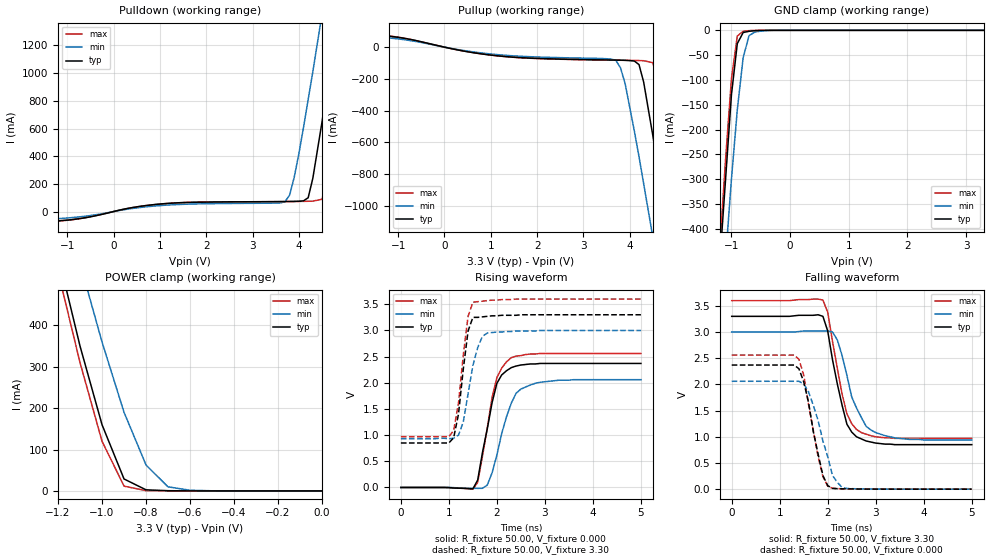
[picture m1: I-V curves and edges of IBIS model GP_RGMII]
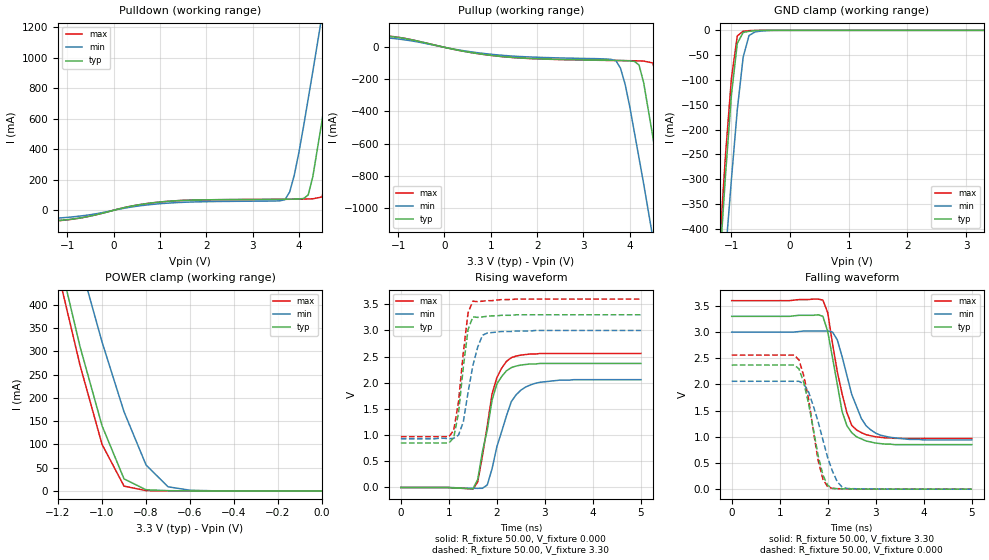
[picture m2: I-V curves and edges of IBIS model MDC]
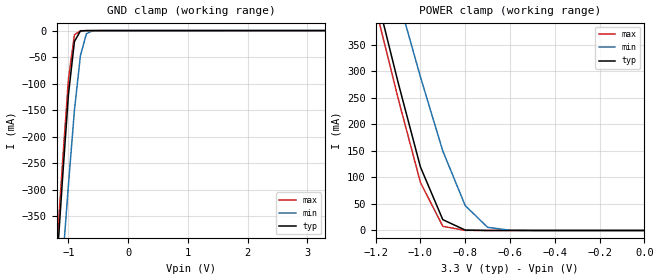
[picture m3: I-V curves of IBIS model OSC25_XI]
|   National Semiconductor Corporation
|   Networks Division
|   IBIS Model for DP83865
|   128 Pin PQFP Package
| IBIS file DP83865.ibs was created using s2ibis2 version 2.1
| North Carolina State University Electronics Research Laboratory 1997
| http://www.eigroup.org/ibis/tools.htm -> SPICE-toIBISconversion(IBISv2.1)
| s2ibis2.tar.Z   11FEB97   652K
| s2ibis2_fix.tar.Z 13MAY97   119K
[IBIS ver]   3.2
[File name]   dp83865.ibs
[File Rev]   1.0
[Date]   07MAY04
[Source]   National Semiconductor Corporation, Networks Division
[Notes]   For questions or comments contact
   jeff.zhang@nsc.com
   Spectre s2ibis simulations, created by Jeff Zhang.
| Due to IBIS modeling limitations and design complexity this model
| does not support the Ethernet Transmit Data pins:
| [Pin]   signal_name   model_name
|108   MDIA_P   NC
|109   MDIA_N   NC
|114   MDIB_P   NC
|115   MDIB_N   NC
|120   MDIC_P   NC
|121   MDIC_N   NC
|126   MDID_P   NC
|127   MDID_N   NC
| Please refer to product datasheet and application notes for PC board
| layout recommendations.
[Disclaimer]  Absolutely no guarantees, for modeling purposes only.
   National Semiconductor Corporation hereby grants the user of this IBIS
model a non-exclusive, nontransferable license to use this IBIS model under
the following terms. Before using this IBIS model, the user should read this
license.  If the user does not accept these terms,  the IBIS model should be
returned to National within 30 days.
   The user is granted this license only to use the IBIS model and is not
granted rights to sell, load, rent, lease or license the IBIS model in whole
or in part, or in modified form to anyone other than user. User may modify
the IBIS model to suit its specific applications but rights to derivative
works and such modifications shall belong to National.
   This IBIS model is provided on an "AS IS" basis and National makes
absolutely no warranty with respect to the information contained herein.
NATIONAL DISCLAIMS AND CUSTOMER WAIVES ALL WARRANTIES, EXPRESS OR IMPLIED,
INCLUDING WARRANTIES OF MERCHANTABILITY OR FITNESS FOR A PARTICULAR PURPOSE.
The entire risk as to quality and performance is with the Customer.
ACCORDINGLY, IN NO EVENT SHALL THE COMPANY BE LIABLE FOR ANY DAMAGES, WHETHER
IN CONTRACT OR COURT, INCLUDING ANY LOST PROFITS OR OTHER INCIDENTAL,
CONSEQUENTIAL, EXEMPLARY, OR PUNITIVE DAMAGES ARISING OUT OF THE USE OR
APPLICATION OF THE IBIS model provided in this package. Further, National
reserves the right to make changes without notice to any product herein to
improve reliability, function, or design. National does not convey any license
under patent rights or any other intellectual property rights, including those
of third parties.
   National is not obligated to provide maintenance or support
for the licensed IBIS model.
[Copyright]   Copyright 2001, National Semiconductor Corporation, All rights
   reserved
|   Component DP83865
[Component]   DP83865
[Manufacturer]   National Semiconductor Corporation
[Package]
| variable   typ   min   max
R_pkg   0.230   0.113   0.305
L_pkg   7.507nH   4.865nH   9.669nH
C_pkg   1.044pF   0.511pF   1.471pF
[Pin]  signal_name   model_name   R_pin   L_pin   C_pin
1   NON_IEEE   GP_RGMII   0.253   9.370nH   1.083pF
2   RESERVED   GP_RGMII   0.255   9.000nH   1.468pF
3   INTERRUPT   GP_RGMII   0.254   8.684nH   1.388pF
4   IO_VDD   POWER   0.255   8.476nH   1.373pF
5   VSS   GND   0.150   6.714nH   1.391pF
6   TX_TCLK   GP_RGMII   0.247   8.104nH   0.756pF
7   ACTIVITY_LED   GP_RGMII   0.246   7.817nH   1.158pF
8   LINK10_LED   GP_RGMII   0.144   6.090nH   1.163pF
9   LINK100_LED   GP_RGMII   0.240   7.452nH   1.064pF
10   AN_EN   GP_RGMII   0.238   7.286nH   1.020pF
11   CORE_VDD   POWER   0.248   7.324nH   0.972pF
12   VSS   GND   0.139   5.513nH   1.007pF
13   PHYADDR0   GP_RGMII   0.241   6.994nH   0.903pF
14   PHYADDR1   GP_RGMII   0.239   6.852nH   0.861pF
15   IO_VDD   POWER   0.236   6.751nH   0.826pF
16   VSS   GND   0.132   5.054nH   0.863pF
17   PHYADDR2   GP_RGMII   0.235   6.563nH   0.771pF
18   PHYADDR3   GP_RGMII   0.235   6.493nH   0.758pF
19   CORE_VDD   POWER   0.236   6.496nH   0.747pF
20   VSS   GND   0.131   4.865nH   0.830pF
21   IO_VDD   POWER   0.234   6.478nH   0.779pF
22   VSS   GND   0.130   4.931nH   0.841pF
23   RESERVED   RGMII125   0.233   6.607nH   0.798pF
24   TCK   RGMII125   0.233   6.664nH   0.510pF
25   CORE_VDD   POWER   0.230   6.679nH   0.854pF
26   VSS   GND   0.131   5.237nH   0.959pF
27   TMS   RGMII125   0.230   6.897nH   0.933pF
28   TDO   RGMII125   0.231   7.040nH   0.965pF
29   IO_VDD   POWER   0.233   7.185nH   1.016pF
30   VSS   GND   0.138   5.850nH   1.124pF
31   TDI   RGMII125   0.237   7.512nH   1.094pF
32   TRST   RGMII125   0.240   7.696nH   1.153pF
33   RESET   RGMII125   0.242   7.992nH   1.236pF
34   VDD_SEL_   POWER   0.249   8.221nH   1.314pF
35   CORE_VDD   POWER   0.255   8.455nH   1.368pF
36   VSS   GND   0.154   7.133nH   1.451pF
37   IO_VDD   POWER   0.255   8.994nH   1.467pF
38   VSS   GND   0.153   7.819nH   1.139pF
39   COL   RGMII125   0.269   9.342nH   0.946pF
40   CRS/RGMII_SEL1 RGMII125   0.263   8.929nH   1.261pF
41   RX_ER   RGMII125   0.259   8.740nH   1.215pF
42   IO_VDD   POWER   0.256   8.546nH   1.164pF
43   VSS   GND   0.146   6.880nH   1.200pF
44   RX_DV   RGMII125   0.257   8.489nH   1.110pF
45   RXD7   RGMII125   0.257   8.359nH   1.082pF
46   RXD6   RGMII125   0.257   8.221nH   1.043pF
47   RXD5   RGMII125   0.259   8.168nH   0.992pF
48   CORE_VDD   POWER   0.261   8.113nH   1.023pF
49   VSS   GND   0.150   6.313nH   1.095pF
50   RXD4   RGMII125   0.268   8.069nH   0.982pF
51   RXD3   RGMII125   0.270   7.874nH   1.019pF
52   RXD2   RGMII125   0.271   7.932nH   1.006pF
53   IO_VDD   POWER   0.266   7.939nH   0.969pF
54   VSS   GND   0.147   6.100nH   1.046pF
55   RXD1   RGMII125   0.260   7.942nH   0.987pF
56   RXD0   RGMII125   0.258   7.994nH   1.009pF
57   RX_CLK   RGMII125   0.258   8.084nH   1.038pF
58   IO_VDD   POWER   0.257   8.189nH   1.069pF
59   VSS   GND   0.147   6.592nH   1.176pF
60   TX_CLK   RGMII125   0.257   8.416nH   1.131pF
61   TX_ER   RGMII125   0.259   8.605nH   1.166pF
62   TX_EN   RGMII125   0.262   8.804nH   1.217pF
63   CORE_VDD   POWER   0.266   9.075nH   1.269pF
64   VSS   GND   0.158   7.609nH   1.020pF
65   TXD7   RGMII125   0.249   9.245nH   1.078pF
66   TXD6   RGMII125   0.251   8.879nH   1.471pF
67   TXD5   RGMII125   0.250   8.587nH   1.388pF
68   TXD4   RGMII125   0.250   8.299nH   1.374pF
69   IO_VDD   POWER   0.245   8.062nH   1.319pF
70   VSS   GND   0.144   6.356nH   1.297pF
71   TXD3   RGMII125   0.238   7.661nH   1.152pF
72   TXD2   RGMII125   0.236   7.480nH   1.092pF
73   CORE_VDD   POWER   0.232   7.306nH   1.059pF
74   VSS   GND   0.135   5.664nH   1.077pF
75   TXD1   RGMII125   0.230   7.022nH   0.964pF
76   TXD0   RGMII125   0.230   6.884nH   0.932pF
77   IO_VDD   POWER   0.234   6.820nH   0.895pF
78   VSS   GND   0.132   5.152nH   0.920pF
79   GTX_CLK   RGMII125   0.234   6.685nH   0.823pF
80   MDIO   MDC   0.234   6.607nH   0.792pF
81   MDC   MDC   0.233   6.528nH   0.770pF
82   VSS   GND   0.234   6.473nH   0.757pF
83   IO_VDD   POWER   0.236   6.484nH   0.747pF
84   RESERVED   RGMII125   0.244   6.522nH   0.764pF
85   CLK_TO_MAC   RGMII125   0.234   6.472nH   0.779pF
86   CLK_IN   OSC25_XI   0.234   6.563nH   0.774pF
87   CLK_OUT   GP_RGMII   0.234   6.659nH   0.800pF
88   MAC_CLK_EN   GP_RGMII   0.234   6.756nH   0.514pF
89   MDIX_EN   GP_RGMII   0.238   6.847nH   0.860pF
90   IO_VDD   POWER   0.239   6.970nH   0.903pF
91   VSS   GND   0.139   5.546nH   1.010pF
92   CORE_VDD   POWER   0.244   7.313nH   0.975pF
93   VSS   GND   0.144   5.860nH   1.094pF
94   MULTI_EN   GP_RGMII   0.244   7.545nH   1.068pF
95   PHYADDR4   GP_RGMII   0.248   7.698nH   1.099pF
96   AFE_VDD   POWER   0.242   7.744nH   1.155pF
97   VSS   GND   0.241   7.925nH   1.237pF
98   PGM_VDD   POWER   0.247   8.077nH   1.314pF
99   VSS   GND   0.250   8.273nH   1.366pF
100   CORE_VDD   POWER   0.251   8.509nH   1.382pF
101   BG_VDD   POWER   0.251   8.799nH   1.464pF
102   BG_REF   POWER   0.247   9.140nH   1.069pF
103   RX_VDD   POWER   0.287   9.669nH   0.956pF
104   VSS   GND   0.280   9.261nH   1.272pF
105   RX_VDD   POWER   0.275   9.149nH   1.222pF
106   VSS   GND   0.270   8.650nH   1.140pF
107   VSS   GND   0.210   7.942nH   1.078pF
108   MDIA_P   NC   0.287   8.392nH   1.028pF
109   MDIA_N   NC   0.285   8.215nH   0.983pF
110   VSS   GND   0.121   6.271nH   1.022pF
111   RX_VDD   POWER   0.286   8.048nH   0.940pF
112   VSS   GND   0.287   7.943nH   0.901pF
113   VSS   GND   0.191   7.185nH   0.874pF
114   MDIB_P   NC   0.292   7.844nH   0.878pF
115   MDIB_N   NC   0.305   7.848nH   0.928pF
116   VSS   GND   0.113   5.862nH   0.962pF
117   RX_VDD   POWER   0.291   7.804nH   0.868pF
118   VSS   GND   0.287   7.791nH   0.897pF
119   VSS   GND   0.189   7.158nH   0.916pF
120   MDIC_P   NC   0.282   7.898nH   0.939pF
121   MDIC_N   NC   0.281   7.966nH   0.968pF
122   VSS   GND   0.117   6.202nH   1.059pF
123   RX_VDD   POWER   0.280   8.214nH   1.022pF
124   VSS   GND   0.282   8.370nH   1.054pF
125   VSS   GND   0.208   7.942nH   1.125pF
126   MDID_P   NC   0.288   8.769nH   1.145pF
127   MDID_N   NC   0.293   9.013nH   1.224pF
128   VSS   GND   0.140   7.489nH   1.013pF
| Models and submodels in the file (4): GP_RGMII (I/O), MDC (I/O), OSC25_XI (Input), RGMII125 (I/O)
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|   Model GP_RGMII
[Model]   GP_RGMII
Model_type   I/O
Polarity   Non-Inverting
Enable   Active-High
Vinl =   0.80V
Vinh =   2.00V
Vmeas =   1.50V
Cref =  20.00pF
Rref = 100.00k
C_comp   5.00pF   5.00pF   5.00pF
[Temperature Range]   25.00   0.14k   0.000
[Voltage Range]   3.30V   3.00V   3.60V
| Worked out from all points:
|   slope of the pulldown table from 0 to 0.495 V, typ, clamps not added: 14.7 ohm
|   slope of the pullup table from 0 to 0.495 V, typ, clamps not added: 17.2 ohm
|   GND clamp passes 1 mA (typ) near -0.62 V on its own axis
|   POWER clamp passes 1 mA (typ) near -0.72 V on its own axis
|   rising waveform, R_fixture 50.00, V_fixture 0.000: 20-80 % time 312ps typ, 381ps min, 304ps max; typ from 0 V to 2.37 V
|   rising waveform, R_fixture 50.00, V_fixture 3.30: 20-80 % time 189ps typ, 258ps min, 195ps max; typ from 0.85 V to 3.3 V
|   falling waveform, R_fixture 50.00, V_fixture 3.30: 20-80 % time 334ps typ, 423ps min, 330ps max; typ from 3.3 V to 0.85 V
|   falling waveform, R_fixture 50.00, V_fixture 0.000: 20-80 % time 308ps typ, 376ps min, 305ps max; typ from 2.37 V to 0 V
[Pulldown]
| voltage   I(typ)   I(min)   I(max)
-3.3V     -89.91mA   -76.56mA   -93.13mA
-1V       -61.93mA   -46.66mA   -63.1mA
1.2V      59.47mA    47.45mA    59.1mA
3.7V      72.36mA    71.01mA    71.87mA
3.9V      73.37mA    250mA      72.58mA
4.2V      100mA      810mA      74.31mA
4.3V      240mA      1.01A      75.21mA
4.5V      650mA      1.43A      88.74mA
4.7V      1.11A      1.86A      390mA
4.9V      1.58A      2.29A      840mA
5.1V      2.07A      2.73A      1.32A
6.6V      5.81A      6.08A      5.12A
[Pullup]
| voltage   I(typ)   I(min)   I(max)
-3.3V     100mA      91.31mA    110mA
-1.5V     79.4mA     67.53mA    81.97mA
1.3V      -58.96mA   -51mA      -59.25mA
3.7V      -81.52mA   -83.17mA   -82.27mA
3.9V      -83.1mA    -230mA     -83.06mA
4.2V      -110mA     -690mA     -84.55mA
4.3V      -220mA     -860mA     -85.63mA
4.5V      -560mA     -1.2A      -97.98mA
4.7V      -940mA     -1.55A     -350mA
4.9V      -1.33A     -1.91A     -720mA
5.1V      -1.73A     -2.27A     -1.12A
6.6V      -4.89A     -5.08A     -4.33A
[GND_clamp]
| voltage   I(typ)   I(min)   I(max)
-3.3V     -4.64A     -4.34A     -4.71A
-1.2V     -470mA     -620mA     -440mA
-1.1V     -300mA     -460mA     -260mA
-1V       -130mA     -300mA     -97.76mA
-900mV    -26.77mA   -160mA     -11.53mA
-800mV    -4.41mA    -54.89mA   -1.88mA
-700mV    -1.97mA    -10.78mA   -630uA
-600mV    -770uA     -3.36mA    -120uA
-500mV    -170uA     -1.53mA    -11.66uA
-200mV    -41.48nA   -16.34uA   -940pA
3.3V      180pA      10.43uA    45.9pA
[POWER_clamp]
| voltage   I(typ)   I(min)   I(max)
-3.3V     5.63A      5.27A      5.71A
-1.2V     570mA      750mA      530mA
-1.1V     350mA      550mA      310mA
-1V       160mA      360mA      120mA
-900mV    28.86mA    190mA      11.54mA
-800mV    2.64mA     62.61mA    730uA
-700mV    550uA      9.86mA     87.59uA
-600mV    98.75uA    1.62mA     9.39uA
0V        180pA      380nA      53.88pA
[Ramp]
| variable   typ   min   max
dV/dt_r   1.92/0.12n   1.74/0.15n   2.09/0.12n
dV/dt_f   1.93/99.31p   1.74/0.12n   2.11/0.10n
R_load = 0.50k
[Rising Waveform]
R_fixture = 50.00
V_fixture = 0.000
V_fixture_min = 0.000
V_fixture_max = 0.000
| time   V(typ)   V(min)   V(max)
0s        1.26nV     480nV      1.01nV
1.5ns     -26.8mV    -15.77mV   -32.46mV
1.6ns     140mV      -17.36mV   96.56mV
1.8ns     1.12V      45.67mV    1.14V
1.9ns     1.62V      280mV      1.72V
2ns       1.99V      620mV      2.1V
2.3ns     2.29V      1.61V      2.48V
2.5ns     2.34V      1.88V      2.52V
2.9ns     2.37V      2.01V      2.56V
5ns       2.37V      2.06V      2.56V
[Rising Waveform]
R_fixture = 50.00
V_fixture = 3.30
V_fixture_min = 3.00
V_fixture_max = 3.60
| time   V(typ)   V(min)   V(max)
0s        850mV      930mV      970mV
1ns       850mV      930mV      970mV
1.1ns     950mV      940mV      1.09V
1.2ns     1.4V       1V         1.61V
1.3ns     2.26V      1.25V      2.53V
1.4ns     2.99V      1.79V      3.27V
1.5ns     3.25V      2.33V      3.54V
1.7ns     3.26V      2.89V      3.56V
1.8ns     3.27V      2.95V      3.57V
5ns       3.3V       3V         3.6V
[Falling Waveform]
R_fixture = 50.00
V_fixture = 3.30
V_fixture_min = 3.00
V_fixture_max = 3.60
| time   V(typ)   V(min)   V(max)
0s        3.3V       3V         3.6V
1.9ns     3.3V       3.02V      3.61V
2ns       3.02V      3.02V      3.38V
2.2ns     2.01V      2.85V      2.31V
2.4ns     1.24V      2.17V      1.44V
2.5ns     1.09V      1.76V      1.25V
2.7ns     960mV      1.37V      1.08V
2.9ns     900mV      1.13V      1.02V
3.4ns     850mV      980mV      970mV
5ns       850mV      940mV      970mV
[Falling Waveform]
R_fixture = 50.00
V_fixture = 0.000
V_fixture_min = 0.000
V_fixture_max = 0.000
| time   V(typ)   V(min)   V(max)
0s        2.37V      2.06V      2.56V
1.4ns     2.3V       2.06V      2.48V
1.5ns     2.05V      2.01V      2.18V
1.6ns     1.66V      1.86V      1.62V
1.8ns     670mV      1.31V      620mV
1.9ns     260mV      920mV      240mV
2ns       67.8mV     620mV      57.17mV
2.1ns     15.64mV    260mV      16.13mV
2.3ns     6.95mV     32.77mV    7.28mV
5ns       -110nV     14.23uV    1.22uV
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|   Model MDC
[Model]   MDC
Model_type   I/O
Polarity   Non-Inverting
Enable   Active-High
Vinl =   0.80V
Vinh =   2.00V
Vmeas =   1.50V
Cref =  20.00pF
Rref = 100.00k
C_comp   5.00pF   5.00pF   5.00pF
[Temperature Range]   25.00   0.14k   0.000
[Voltage Range]   3.30V   3.00V   3.60V
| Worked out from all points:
|   slope of the pulldown table from 0 to 0.495 V, typ, clamps not added: 14.7 ohm
|   slope of the pullup table from 0 to 0.495 V, typ, clamps not added: 17.2 ohm
|   GND clamp passes 1 mA (typ) near -0.62 V on its own axis
|   POWER clamp passes 1 mA (typ) near -0.72 V on its own axis
|   rising waveform, R_fixture 50.00, V_fixture 0.000: 20-80 % time 313ps typ, 394ps min, 302ps max; typ from 0 V to 2.37 V
|   rising waveform, R_fixture 50.00, V_fixture 3.30: 20-80 % time 188ps typ, 257ps min, 190ps max; typ from 0.85 V to 3.3 V
|   falling waveform, R_fixture 50.00, V_fixture 3.30: 20-80 % time 312ps typ, 417ps min, 340ps max; typ from 3.3 V to 0.85 V
|   falling waveform, R_fixture 50.00, V_fixture 0.000: 20-80 % time 309ps typ, 394ps min, 283ps max; typ from 2.37 V to 0 V
[Pulldown]
| voltage   I(typ)   I(min)   I(max)
-3.3V     -89.91mA   -76.56mA   -93.13mA
-1V       -61.93mA   -46.66mA   -63.1mA
1.2V      59.47mA    47.45mA    59.1mA
3.7V      72.36mA    69.99mA    71.87mA
3.9V      73.37mA    230mA      72.58mA
4.2V      100mA      730mA      74.31mA
4.3V      220mA      910mA      75.21mA
4.5V      590mA      1.28A      87.5mA
4.7V      1A         1.66A      350mA
4.9V      1.42A      2.04A      760mA
5.1V      1.85A      2.43A      1.19A
6.6V      5.19A      5.43A      4.58A
[Pullup]
| voltage   I(typ)   I(min)   I(max)
-3.3V     100mA      91.31mA    110mA
-1.5V     79.4mA     67.53mA    81.97mA
1.3V      -58.96mA   -51mA      -59.25mA
3.7V      -81.52mA   -82.85mA   -82.27mA
3.9V      -83.1mA    -230mA     -83.06mA
4.2V      -110mA     -690mA     -84.55mA
4.3V      -220mA     -850mA     -85.62mA
4.5V      -560mA     -1.19A     -97.65mA
4.7V      -930mA     -1.54A     -340mA
4.9V      -1.32A     -1.89A     -720mA
5.1V      -1.71A     -2.25A     -1.11A
6.6V      -4.85A     -5.04A     -4.3A
[GND_clamp]
| voltage   I(typ)   I(min)   I(max)
-3.3V     -4.6A      -4.3A      -4.67A
-1.2V     -470mA     -610mA     -430mA
-1.1V     -290mA     -450mA     -250mA
-1V       -130mA     -300mA     -96.48mA
-900mV    -26.18mA   -160mA     -11.2mA
-800mV    -4.33mA    -53.85mA   -1.86mA
-700mV    -1.97mA    -10.45mA   -630uA
-600mV    -770uA     -3.3mA     -120uA
-500mV    -170uA     -1.53mA    -11.66uA
-200mV    -41.47nA   -16.34uA   -920pA
3.3V      170pA      10.38uA    37.9pA
[POWER_clamp]
| voltage   I(typ)   I(min)   I(max)
-3.3V     5.01A      4.69A      5.08A
-1.2V     510mA      660mA      470mA
-1.1V     310mA      490mA      270mA
-1V       140mA      320mA      100mA
-900mV    25.8mA     170mA      10.3mA
-800mV    2.47mA     55.78mA    680uA
-700mV    550uA      8.85mA     86.56uA
-600mV    98.6uA     1.5mA      9.37uA
0V        170pA      380nA      44.23pA
[Ramp]
| variable   typ   min   max
dV/dt_r   1.92/0.11n   1.74/0.14n   2.09/0.11n
dV/dt_f   1.93/93.44p   1.74/0.12n   2.11/95.48p
R_load = 0.50k
[Rising Waveform]
R_fixture = 50.00
V_fixture = 0.000
V_fixture_min = 0.000
V_fixture_max = 0.000
| time   V(typ)   V(min)   V(max)
0s        1.14nV     480nV      920pV
1.5ns     -26.61mV   -15.8mV    -32.48mV
1.6ns     150mV      -17.39mV   100mV
1.8ns     1.1V       47.88mV    1.18V
1.9ns     1.67V      360mV      1.79V
2ns       1.98V      780mV      2.1V
2.3ns     2.29V      1.64V      2.48V
2.5ns     2.34V      1.86V      2.53V
2.9ns     2.37V      2.01V      2.56V
5ns       2.37V      2.06V      2.56V
[Rising Waveform]
R_fixture = 50.00
V_fixture = 3.30
V_fixture_min = 3.00
V_fixture_max = 3.60
| time   V(typ)   V(min)   V(max)
0s        850mV      930mV      970mV
1ns       850mV      930mV      970mV
1.1ns     950mV      940mV      1.09V
1.2ns     1.42V      1V         1.63V
1.3ns     2.29V      1.25V      2.57V
1.4ns     3.02V      1.82V      3.34V
1.5ns     3.26V      2.33V      3.56V
1.7ns     3.26V      2.91V      3.56V
1.8ns     3.27V      2.95V      3.57V
5ns       3.3V       3V         3.6V
[Falling Waveform]
R_fixture = 50.00
V_fixture = 3.30
V_fixture_min = 3.00
V_fixture_max = 3.60
| time   V(typ)   V(min)   V(max)
0s        3.3V       3V         3.6V
1.9ns     3.3V       3.02V      3.61V
2ns       3.01V      3.02V      3.37V
2.1ns     2.51V      3V         2.78V
2.3ns     1.48V      2.53V      1.82V
2.5ns     1.08V      1.81V      1.22V
2.6ns     1V         1.58V      1.13V
2.8ns     920mV      1.21V      1.04V
3.1ns     870mV      1.03V      990mV
5ns       850mV      940mV      970mV
[Falling Waveform]
R_fixture = 50.00
V_fixture = 0.000
V_fixture_min = 0.000
V_fixture_max = 0.000
| time   V(typ)   V(min)   V(max)
0s        2.37V      2.06V      2.56V
1.3ns     2.37V      2.06V      2.56V
1.4ns     2.3V       2.06V      2.47V
1.6ns     1.64V      1.86V      1.73V
1.8ns     640mV      1.29V      550mV
1.9ns     270mV      940mV      190mV
2ns       72.26mV    600mV      41.72mV
2.2ns     9.3mV      140mV      9.26mV
2.4ns     5.17mV     14.05mV    5.01mV
5ns       -13.03uV   18.75uV    -80.37nV
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|   Model OSC25_XI
[Model]   OSC25_XI
Model_type   Input
Polarity   Non-Inverting
Enable   Active-Low
Vinl =   0.80V
Vinh =   2.00V
Vmeas =   1.50V
Cref =  10.00pF
Rref = 100.00k
C_comp   5.00pF   5.00pF   5.00pF
[Temperature Range]   25.00   0.14k   0.000
[Voltage Range]   3.30V   3.00V   3.60V
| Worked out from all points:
|   GND clamp passes 1 mA (typ) near -0.80 V on its own axis
|   POWER clamp passes 1 mA (typ) near -0.80 V on its own axis
[GND_clamp]
| voltage   I(typ)   I(min)   I(max)
-3.3V     -4.5A      -4.21A     -4.58A
-1.2V     -450mA     -600mA     -420mA
-1.1V     -280mA     -440mA     -250mA
-1V       -120mA     -290mA     -91.03mA
-900mV    -20.53mA   -150mA     -8mA
-800mV    -820uA     -47.26mA   -220uA
-700mV    -49.04uA   -6.03mA    -19.31uA
-600mV    -11.96uA   -550uA     -9.05uA
3.3V      8.24uA     10.27uA    6.92uA
[POWER_clamp]
| voltage   I(typ)   I(min)   I(max)
-3.3V     4.5A       4.21A      4.58A
-1.2V     450mA      600mA      420mA
-1.1V     280mA      440mA      250mA
-1V       120mA      290mA      90.87mA
-900mV    20.41mA    150mA      7.91mA
-800mV    760uA      47.07mA    190uA
-700mV    29.01uA    5.92mA     11.87uA
-600mV    10.15uA    490uA      8.85uA
0V        8.24uA     9.21uA     7.55uA
